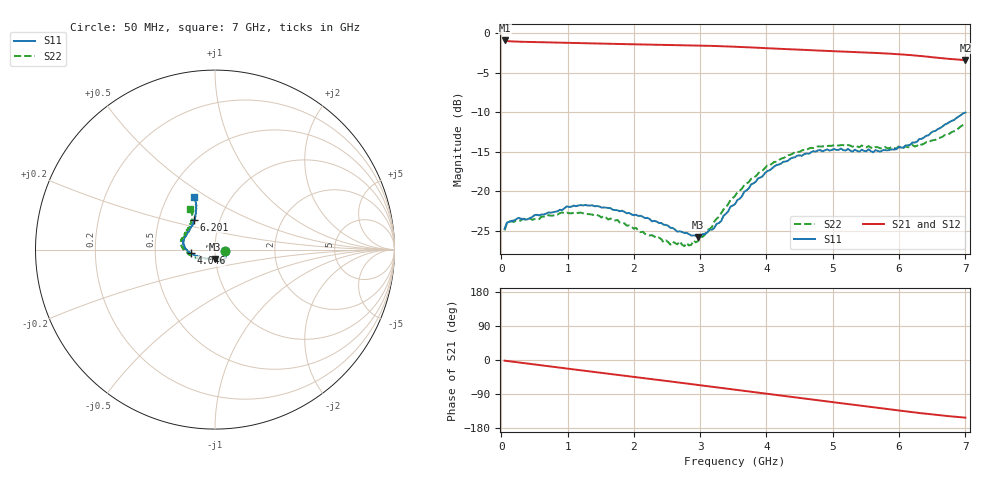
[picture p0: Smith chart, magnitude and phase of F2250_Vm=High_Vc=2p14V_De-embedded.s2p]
! Integrated Device Technology
! Corporate Headquarters
! 6024 Silver Creek Valley Road
! San Jose, CA 95138  USA
! Phone:  1-408-284-8200
! Toll Free:  1-800-223-1366
! Webpage:  http://www.idt.com/
! Timing and RF Division
! 515 Groton Road, Suite 102
! Westford, MA 01886-6024
! Device:  F2250
! Description: Voltage Variable RF Attenuator
! Frequency:  50.0 -  6000.00 MHz
! Package:  3x3 mm Thin QFN Plastic Package: 16 pin
! Ports:  2 RF, 3 DC
!  Pin  1  = GND
!  Pin  2  = NC
!  Pin  3  = RF1  = Port 1
!  Pin  4  = NC
!  Pin  5  = GND
!  Pin  6  = GND
!  Pin  7  = GND
!  Pin  8  = GND
!  Pin  9  = NC
!  Pin 10  = RF2  = Port 2
!  Pin 11  = NC
!  Pin 12  = GND
!  Pin 13  = GND
!  Pin 14  = VCNTRL
!  Pin 15  = VDD
!  Pin 16  = VMODE
! Vcntrl:  2.140 Volts
! Vmode:  +3.300 Volts
! Vdd:  +3.30  Volts
! Current:  1.317 mA
! Data:  The device was measured on a the F2250 evaluation board which has
!  individual transmission lines to the RF pins.  Data was collected
!  using a calibrated network analyzer.  The evaluation board was
!  de-embedded using a TRL calibration technique.
!  The reference plane is the edge of the package pin.
! Misc:  SN 10
!  Action Tracker AT0258
! Date Measured:  2014-11-26
! Date:  2015-10-15  MJV
! Note:
!  Integrated Device Technology supplies this data as a sample of measured
!  data at the package pin for this product.  Your particular data for this
!  product may vary.
!  Data was taken at 25 degrees C.
!  Integrated Device Technology reserves the right to change this data at anytime.
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# GHz S dB R 50
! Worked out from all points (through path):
!   201 points, 50 MHz to 7 GHz, reference 50 ohm
!   highest |S21| = -0.95 dB at 50 MHz (marker M1); lowest = -3.4 dB at 7 GHz (marker M2)
!   group delay of S21, straight-line fit = 61.1 ps
!   lowest |S11| = -25.7 dB at 2.969 GHz (marker M3), VSWR 1.11, Z = 49.5 - j5.13 ohm
!   |S11| at or under -10 dB: start of sweep to end of sweep
!   |S22| runs from -26.9 to -11.5 dB; largest |S21 - S12| = 0.0019
!   S11 on the Smith chart (normalised r, x): 50 MHz: 1.12, -0.02; 4.046 GHz: 0.76, -0.03; 6.201 GHz: 0.75, +0.26; 7 GHz: 0.68, +0.44
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0.05  -24.73 -9.6  -0.95 -1.8  -0.95 -1.8  -24.91 -10.1
0.08475  -23.94 -8.8  -1.02 -2.5  -1.02 -2.5  -24.01 -9.0
0.1195  -23.83 -9.4  -1.05 -3.3  -1.05 -3.2  -23.82 -8.4
0.91875  -22.35 -47.2  -1.24 -21.0  -1.23 -21.1  -22.64 -49.2
1.2315  -21.77 -55.0  -1.30 -27.9  -1.30 -27.9  -22.76 -59.7
1.75275  -22.38 -61.8  -1.39 -39.1  -1.39 -39.1  -23.59 -66.8
2.37825  -23.98 -62.0  -1.49 -52.8  -1.49 -52.8  -25.83 -68.3
2.552  -24.60 -66.5  -1.51 -56.6  -1.51 -56.7  -26.72 -74.9
2.691  -25.02 -73.8  -1.53 -59.7  -1.53 -59.7  -26.31 -82.1
2.7605  -25.25 -75.8  -1.55 -61.3  -1.55 -61.3  -26.91 -86.5
2.969  -25.73 -92.4  -1.59 -66.0  -1.59 -66.0  -26.26 -104.6
3.21225  -24.63 -121.9  -1.64 -71.4  -1.64 -71.5  -23.82 -128.7
3.525  -21.62 -148.4  -1.74 -78.5  -1.74 -78.5  -20.57 -147.4
3.76825  -19.11 -161.6  -1.83 -84.0  -1.83 -84.0  -18.41 -158.6
4.04625  -17.33 -171.5  -1.94 -90.2  -1.94 -90.2  -16.73 -169.1
4.4285  -15.69 178.0  -2.09 -98.6  -2.10 -98.6  -15.03 179.4
4.7065  -14.92 170.9  -2.19 -104.8  -2.19 -104.8  -14.53 173.6
5.054  -14.77 162.6  -2.32 -112.4  -2.31 -112.5  -14.14 166.4
5.85325  -14.78 136.6  -2.62 -130.0  -2.62 -130.1  -14.55 147.6
6.20075  -13.83 124.8  -2.82 -137.7  -2.83 -137.8  -14.15 138.5
6.54825  -12.37 116.5  -3.10 -144.7  -3.10 -144.8  -13.49 127.1
7  -10.05 111.5  -3.42 -152.0  -3.43 -152.2  -11.49 120.8
